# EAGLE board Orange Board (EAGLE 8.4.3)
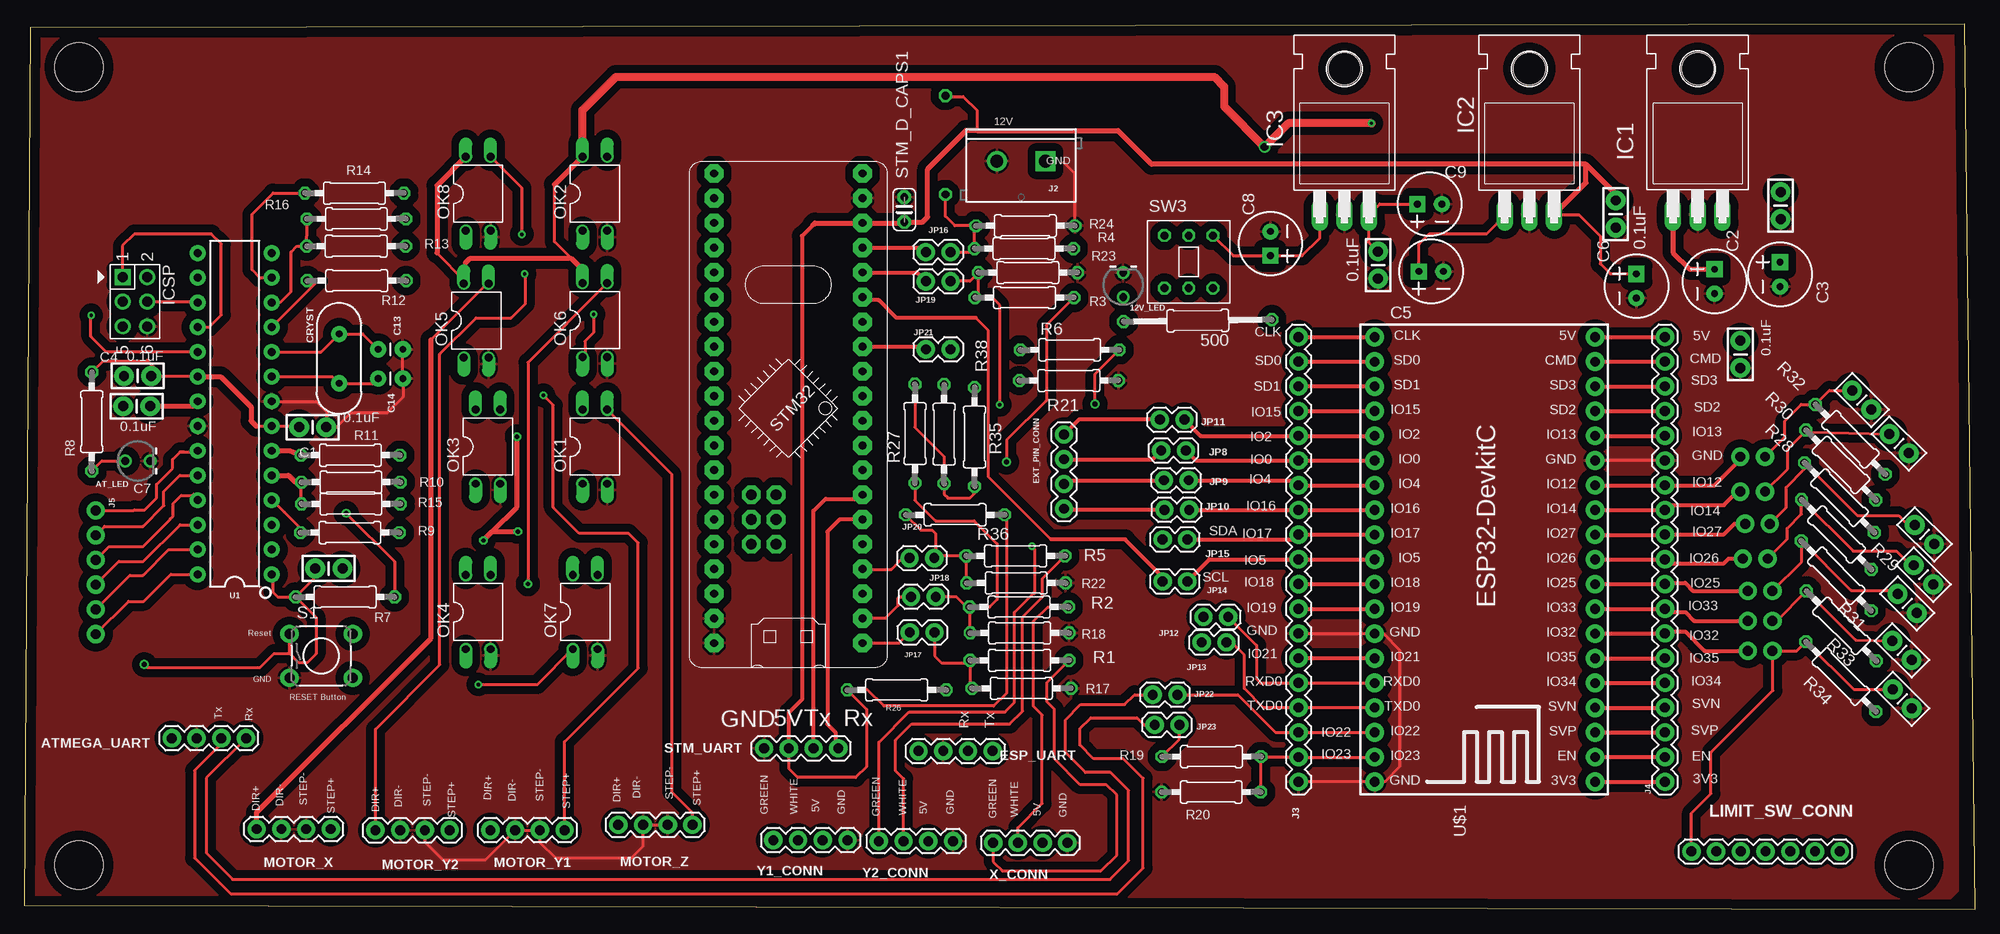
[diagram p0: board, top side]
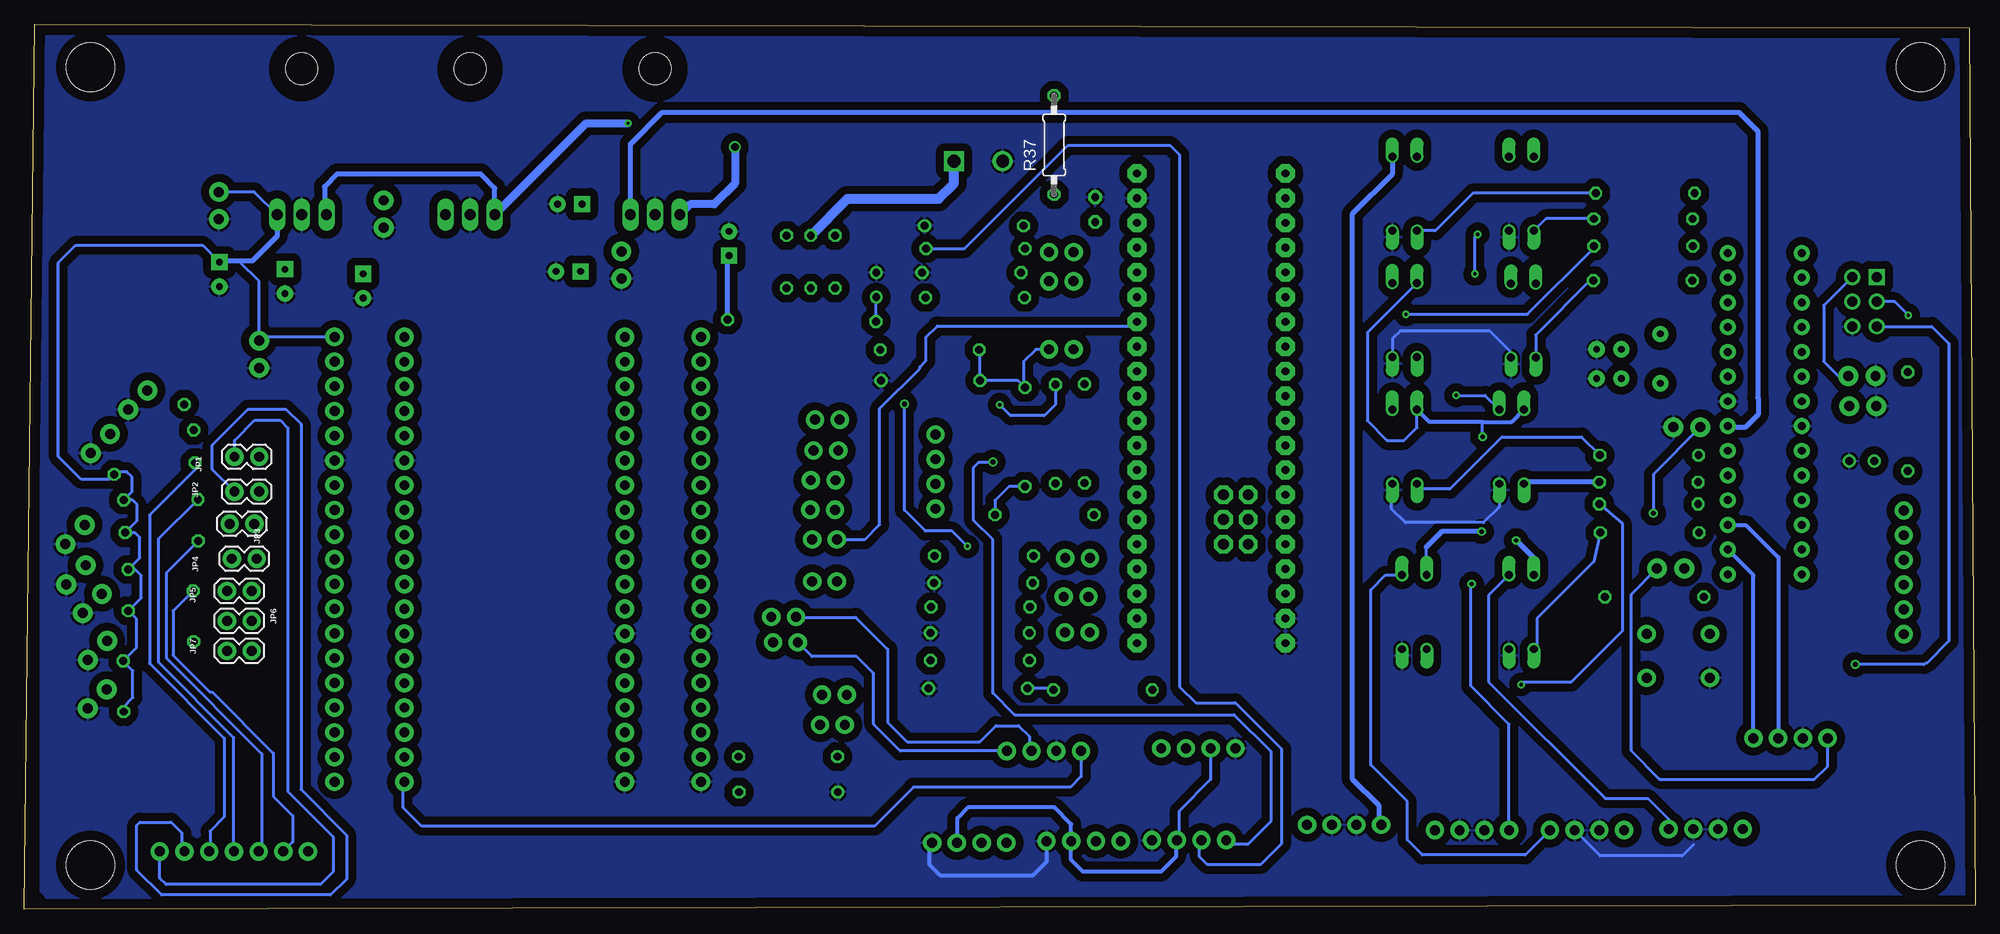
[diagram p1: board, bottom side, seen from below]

Size 200.42 x 90.95 mm. Coordinates in mm from the lower left corner, seen from the top.
Outline: 0,0.41 200.42,0 199.36,90.95 0.6,90.58 0,0.41
Copper layers (1*16): Top 0.035mm / dielectric 1.5mm / Bottom 0.035mm
Design rules "default *": minimum track width 12mil, minimum drill 0.35mm, track to track 12mil, track to pad 12mil, pad to pad 12mil, via to via 12mil, smd to smd 6mil, copper to edge 40mil, drill to drill 12mil, minimum pad ring 10mil, minimum via ring 8mil, stop-mask expansion 4mil, vias tented up to drill 0mil, thermal gap 10mil
Holes 5 mm at 5.62,86.55 193.62,86.55 5.62,4.55 193.62,4.55

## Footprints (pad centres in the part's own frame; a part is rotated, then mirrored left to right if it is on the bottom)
LED_3MM-NS = drill 0.813: A -1.27,0; K 1.27,0
0207/15 = drill 0.813 octagon: 1 -7.62,0; 2 7.62,0
1X04 = drill 1.016 pad 1.88: 1 0,0; 2 2.54,0; 3 5.08,0; 4 7.62,0
CAP-PTH-SMALL-KIT = drill 1.016 pad 2.032: 1 -1.397,0; 2 1.397,0
CPOL-RADIAL-2.5MM-6.5MM = drill 0.7 pad 1.651 square: 1 1.25,0 | drill 0.7 pad 1.651: 2 -1.25,0
CAP-PTH-2.54 = drill 0.7 pad 1.651: 1 -1.27,0; 2 1.27,0
HC49US = drill 0.7 pad 1.651: 1 -2.54,0; 2 2.54,0
TO220H = drill 1.118 long: 1 -2.54,-10.16; 2 0,-10.16; 3 2.54,-10.16 | hole 3.302: 0,4.826
HEADER_PRG_2X03 = drill 1.02 pad 1.632 square: 1 -2.54,-1.27 | drill 1.02 pad 1.632: 2 -2.54,1.27; 3 0,-1.27; 4 0,1.27; 5 2.54,-1.27; 6 2.54,1.27
SCREWTERMINAL-5MM-2 = drill 1.3 pad 2.032 square: 1 0,0 | drill 1.3 pad 2.032: 2 5,0
1X19 = drill 1.016 pad 1.88: 1 0,0; 2 2.54,0; 3 5.08,0; 4 7.62,0; 5 10.16,0; 6 12.7,0; 7 15.24,0; 8 17.78,0; 9 20.32,0; 10 22.86,0; 11 25.4,0; 12 27.94,0; 13 30.48,0; 14 33.02,0; 15 35.56,0; 16 38.1,0; 17 40.64,0; 18 43.18,0; 19 45.72,0
1X06_NO_SILK = drill 1.016 pad 1.88: 1 0,0; 2 2.54,0; 3 5.08,0; 4 7.62,0; 5 10.16,0; 6 12.7,0
1X02 = drill 1.016 pad 1.88: 1 0,0; 2 2.54,0
1X07 = drill 1.016 pad 1.88: 1 0,0; 2 2.54,0; 3 5.08,0; 4 7.62,0; 5 10.16,0; 6 12.7,0; 7 15.24,0
DIL04 = drill 0.813 offset: 1 -1.27,-3.81; 2 1.27,-3.81; 3 1.27,3.81; 4 -1.27,3.81
0207/10 = drill 0.813 octagon: 1 -5.08,0; 2 5.08,0
TACTILE-PTH = drill 1.016 pad 1.88: 1 -3.251,2.261; 2 3.251,2.261; 3 -3.251,-2.261; 4 3.251,-2.261
C025-024X044 = drill 0.813 pad 1.422 octagon: 1 -1.27,0; 2 1.27,0
SW_PUSH_BUTTON_MINI = drill 0.8 octagon: 1 2.5,2.7; 2 0,2.7; 3 -2.5,2.7; 4 2.5,-2.7; 5 0,-2.7; 6 -2.5,-2.7
DIP28 = drill 0.813 pad 1.626: 1 -16.51,-3.81; 2 -13.97,-3.81; 3 -11.43,-3.81; 4 -8.89,-3.81; 5 -6.35,-3.81; 6 -3.81,-3.81; 7 -1.27,-3.81; 8 1.27,-3.81; 9 3.81,-3.81; 10 6.35,-3.81; 11 8.89,-3.81; 12 11.43,-3.81; 13 13.97,-3.81; 14 16.51,-3.81; 15 16.51,3.81; 16 13.97,3.81; 17 11.43,3.81; 18 8.89,3.81; 19 6.35,3.81; 20 3.81,3.81; 21 1.27,3.81; 22 -1.27,3.81; 23 -3.81,3.81; 24 -6.35,3.81; 25 -8.89,3.81; 26 -11.43,3.81; 27 -13.97,3.81; 28 -16.51,3.81
ESP32-DEVKITC = drill 1 pad 1.93: 1 -22.87,-11.42; 2 -20.33,-11.42; 3 -17.79,-11.42; 4 -15.25,-11.42; 5 -12.71,-11.42; 6 -10.17,-11.42; 7 -7.63,-11.42; 8 -5.09,-11.42; 9 -2.55,-11.42; 10 -0.01,-11.42; 11 2.53,-11.42; 12 5.07,-11.42; 13 7.61,-11.42; 14 10.15,-11.42; 15 12.69,-11.42; 16 15.23,-11.42; 17 17.77,-11.42; 18 20.31,-11.42; 19 22.85,-11.42; 20 22.85,11.23; 21 20.31,11.23; 22 17.77,11.23; 23 15.23,11.23; 24 12.69,11.23; 25 10.15,11.23; 26 7.61,11.23; 27 5.07,11.23; 28 2.53,11.23; 29 -0.01,11.23; 30 -2.55,11.23; 31 -5.09,11.23; 32 -7.63,11.23; 33 -10.17,11.23; 34 -12.71,11.23; 35 -15.25,11.23; 36 -17.79,11.23; 37 -20.33,11.23; 38 -22.87,11.23
BLUE_PILL_ADV = drill 0.8 pad 1.93 octagon: P$1 10.16,-30.48; P$2 10.16,-27.94; P$3 10.16,-25.4; P$4 10.16,-22.86; P$5 10.16,-20.32; P$6 10.16,-17.78; P$7 10.16,-15.24; P$8 10.16,-12.7; P$9 10.16,-10.16; P$10 10.16,-7.62; P$11 10.16,-5.08; P$12 10.16,-2.54; P$13 10.16,0; P$14 10.16,2.54; P$15 10.16,5.08; P$16 10.16,7.62; P$17 10.16,10.16; P$18 10.16,12.7; P$19 10.16,15.24; P$20 10.16,17.78; P$21 -5.08,-30.48; P$22 -5.08,-27.94; P$23 -5.08,-25.4; P$24 -5.08,-22.86; P$25 -5.08,-20.32; P$26 -5.08,-17.78; P$27 -5.08,-15.24; P$28 -5.08,-12.7; P$29 -5.08,-10.16; P$30 -5.08,-7.62; P$31 -5.08,-5.08; P$32 -5.08,-2.54; P$33 -5.08,0; P$34 -5.08,2.54; P$35 -5.08,5.08; P$36 -5.08,7.62; P$37 -5.08,10.16; P$38 -5.08,12.7; P$39 -5.08,15.24; P$40 -5.08,17.78 | drill 1.1 pad 1.93 octagon: P$42 -1.27,-20.32; P$43 -1.27,-17.78; P$44 -1.27,-15.24; P$45 1.27,-15.24; P$46 1.27,-17.78; P$47 1.27,-20.32

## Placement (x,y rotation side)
12V_LED  [LED_3MM-NS]  112.9,64.18 90 top
500  1K  [0207/15]  120.55,60.5 180.7 top
AT_LED  [LED_3MM-NS]  11.65,46.08 0 top
ATMEGA_UART  [1X04]  22.78,17.59 180 top
C1  0.1uF  [CAP-PTH-SMALL-KIT]  29.62,49.55 0 top
C2  100uF  [CPOL-RADIAL-2.5MM-6.5MM]  173.65,64.53 90 top
C3  100uF  [CPOL-RADIAL-2.5MM-6.5MM]  180.38,65.25 90 top
C4  0.1uF  [CAP-PTH-SMALL-KIT]  11.63,54.82 180 top
C5  100uF  [CPOL-RADIAL-2.5MM-6.5MM]  144.53,65.56 180 top
C6  100uF  [CPOL-RADIAL-2.5MM-6.5MM]  165.63,64.06 90 top
C7  0.1uF  [CAP-PTH-SMALL-KIT]  11.55,51.71 180 top
C8  100uF  [CPOL-RADIAL-2.5MM-6.5MM]  128.01,68.42 270 top
C9  100uF  [CPOL-RADIAL-2.5MM-6.5MM]  144.38,72.47 180 top
C10  0.1uF  [CAP-PTH-SMALL-KIT]  180.44,72.33 270 top
C11  0.1uF  [CAP-PTH-SMALL-KIT]  163.49,71.45 270 top
C12  0.1uF  [CAP-PTH-SMALL-KIT]  139.08,66.21 270 top
C13  22pF  [CAP-PTH-2.54]  37.62,57.55 180 top
C14  22pF  [CAP-PTH-2.54]  37.62,54.55 180 top
C15  0.1uF  [CAP-PTH-SMALL-KIT]  31.29,35.02 0 top
C18  0.1uF  [CAP-PTH-SMALL-KIT]  195.22,38.52 135 top
C19  0.1uF  [CAP-PTH-SMALL-KIT]  195.12,34.38 135 top
C20  0.1uF  [CAP-PTH-SMALL-KIT]  192.6,47.87 135 top
C21  0.1uF  [CAP-PTH-SMALL-KIT]  193.44,31.43 135 top
C22  0.1uF  [CAP-PTH-SMALL-KIT]  188.77,52.34 135 top
C23  0.1uF  [CAP-PTH-SMALL-KIT]  192.91,26.61 135 top
C24  0.1uF  [CAP-PTH-SMALL-KIT]  192.93,21.63 135 top
CRYST  16MHz  [HC49US]  32.33,56.6 270 top
ESP_D_CAPS  0.1uF  [CAP-PTH-SMALL-KIT]  176.3,57.04 270 top
ESP_UART  [1X04]  99.48,16.27 180 top
EXT_PIN_CONN  [1X04]  106.81,41.17 90 top
IC1  7805T  [TO220H]  171.92,81.56 0 top
IC2  7805T  [TO220H]  154.62,81.55 0 top
IC3  7805T  [TO220H]  135.62,81.55 0 top
ICSP  CON_HEADER_PRG_AVR_ICSP-PTH  [HEADER_PRG_2X03]  11.36,62.45 270 top
J2  [SCREWTERMINAL-5MM-2]  104.92,76.89 180 top
J3  [1X19]  130.91,13.11 90 top
J4  [1X19]  168.55,13.11 90 top
J5  [1X06_NO_SILK]  7.33,40.99 270 top
JP1  [1X02]  176.29,46.51 180 bottom
JP2  [1X02]  176.29,42.93 180 bottom
JP3  [1X02]  176.79,39.62 180 bottom
JP4  [1X02]  176.56,36.04 180 bottom
JP5  [1X02]  177.06,32.73 180 bottom
JP6  [1X02]  177.06,29.65 180 bottom
JP7  [1X02]  177.06,26.57 180 bottom
JP8  [1X02]  119.34,47.16 180 top
JP9  [1X02]  119.62,44.09 180 top
JP10  [1X02]  119.67,41.06 180 top
JP11  [1X02]  119.19,50.32 180 top
JP12  [1X02]  123.68,30.05 180 top
JP13  [1X02]  123.5,27.44 180 top
JP14  [1X02]  119.48,33.7 180 top
JP15  [1X02]  119.48,38.01 180 top
JP16  [1X02]  92.62,67.55 0 top
JP17  [1X02]  90.97,28.45 0 top
JP18  [1X02]  91.1,32.12 0 top
JP19  [1X02]  92.62,64.55 0 top
JP20  [1X02]  90.94,36.1 0 top
JP21  [1X02]  92.62,57.55 0 top
JP22  [1X02]  118.47,22.06 180 top
JP23  [1X02]  118.67,18.96 180 top
LIMIT_SW_CONN  [1X07]  186.51,5.95 180 top
MOTOR_X  [1X04]  31.49,8.25 180 top
MOTOR_Y1  [1X04]  55.5,8.14 180 top
MOTOR_Y2  [1X04]  43.69,8.13 180 top
MOTOR_Z  [1X04]  68.64,8.69 180 top
OK1  PC817  [DIL04]  58.62,47.55 0 top
OK2  PC817  [DIL04]  58.62,73.55 0 top
OK3  PC817  [DIL04]  47.62,47.55 0 top
OK4  PC817  [DIL04]  46.62,30.55 0 top
OK5  PC817  [DIL04]  46.42,60.51 0 top
OK6  PC817  [DIL04]  58.62,60.55 0 top
OK7  PC817  [DIL04]  57.62,30.55 0 top
OK8  PC817  [DIL04]  46.62,73.55 0 top
R1  1K  [0207/10]  102.25,25.58 0 top
R2  1K  [0207/10]  102.19,31.07 0 top
R3  1K  [0207/10]  102.75,62.87 0 top
R4  1K  [0207/10]  102.7,67.91 0 top
R5  1K  [0207/10]  101.84,36.33 0 top
R6  1K  [0207/10]  107.4,57.5 0 top
R7  1K  [0207/10]  32.95,32.11 0 top
R8  1K  [0207/10]  6.93,50.12 270 top
R9  1K  [0207/10]  33.44,38.71 0 top
R10  1K  [0207/10]  33.55,43.9 0 top
R11  1K  [0207/10]  33.5,46.67 0 top
R12  1K  [0207/10]  34.15,64.61 0 top
R13  1K  [0207/10]  34.09,68.15 0 top
R14  1K  [0207/10]  33.91,73.61 0 top
R15  1K  [0207/10]  33.55,41.66 0 top
R16  1K  [0207/10]  34.11,70.96 0 top
R17  2K  [0207/10]  102.43,22.71 180 top
R18  2K  [0207/10]  102.25,28.41 180 top
R19  1K  [0207/10]  121.97,15.7 0 top
R20  1K  [0207/10]  121.93,12.05 180 top
R21  2K  [0207/10]  107.32,54.35 180 top
R22  2K  [0207/10]  101.9,33.53 180 top
R23  2K  [0207/10]  103.1,65.44 180 top
R24  2K  [0207/10]  102.84,70.24 180 top
R26  1K  [0207/10]  89.62,22.55 180 top
R27  1K  [0207/10]  91.5,48.89 90 top
R28  [0207/10]  186.48,42.31 135 top
R29  [0207/10]  186.17,38.52 135 top
R30  [0207/10]  186.63,45.66 135 top
R31  [0207/10]  186.15,34.28 135 top
R32  [0207/10]  187.6,48.3 135 top
R33  [0207/10]  186.68,29.12 135 top
R34  [0207/10]  186.63,23.92 135 top
R35  1K  [0207/10]  97.62,48.55 270 top
R36  1K  [0207/10]  95.62,40.55 0 top
R37  1K  [0207/10]  94.62,78.55 90 bottom
R38  1K  [0207/10]  94.5,48.84 270 top
S1  [TACTILE-PTH]  30.5,26.05 0 top
STM_D_CAPS1  0.1uF  [C025-024X044]  90.41,71.91 90 top
STM_UART  [1X04]  83.62,16.55 180 top
SW3  SW_PUSH_DPDT  [SW_PUSH_BUTTON_MINI]  119.62,66.55 0 top
U1  328P  [DIP28]  21.61,50.94 90 top
U$1  ESP32DEVKITC  [ESP32-DEVKITC]  149.96,35.97 90 top
U$2  [BLUE_PILL_ADV]  75.95,57.84 0 top
X_CONN  [1X04]  99.53,6.84 0 top
Y1_CONN  [1X04]  76.94,7.11 0 top
Y2_CONN  [1X04]  87.79,7.01 0 top

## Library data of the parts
12V_LED AT_LED = SparkFun-LED
500 R1-R24 R26-R38 = resistor
ATMEGA_UART ESP_UART EXT_PIN_CONN MOTOR_X MOTOR_Y1 MOTOR_Y2 MOTOR_Z STM_UART X_CONN Y1_CONN Y2_CONN = SparkFun-Connectors; PROD_ID: CONN-09696
C1 C4 C7 C10-C12 C15 C18-C24 ESP_D_CAPS = SparkFun-Capacitors; PROD_ID: CAP-08370
C2 C3 C5 C6 C8 C9 = SparkFun-Capacitors; PROD_ID: CAP-08439
C13 C14 = SparkFun-Capacitors; PROD_ID: CAP-09128
CRYST = SparkFun-Clocks; PROD_ID: XTAL-08181; SF_ID: COM-00536
IC1-IC3 STM_D_CAPS1 = adafruit
ICSP SW3 = dp_devices
J2 = SparkFun-Connectors; SF_SKU: PRT-08432
J3 J4 LIMIT_SW_CONN = SparkFun-Connectors
J5 = SparkFun-Connectors; PROD_ID: CONN-08437
JP1-JP23 S1 = SparkFun-Retired
OK1-OK8 = optocoupler; MPN: PC817X4J000F; OC_FARNELL: 9707727; OC_NEWARK: 97K7059
U1 = SparkFun-IC-Microcontroller; PROD_ID: IC-09136
U$1 = ESP32-DEVKITC
U$2 = BluePill

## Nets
3V3: ESP_UART.4 J4.1 U$1.1
12V: J2.1 SW3.2
12V_SIN: 500.1 C2.1 C5.1 C8.1 IC1.1 IC2.1 IC3.1 OK1.4 OK2.4 OK3.4 OK4.4 OK5.4 OK6.4 OK7.4 OK8.4 SW3.1
A0: J5.1 U1.23
A1: J5.2 U1.24
A2: J5.3 U1.25
A3: J5.4 U1.26
A4: J5.5 U1.27
A5: J5.6 U1.28
AT_5V: C1.1 C4.1 C9.1 C12.1 IC3.3 ICSP.2 R7.2 R8.1 U1.7 U1.20
AT_JRX: ATMEGA_UART.1 JP22.2 U1.2
AT_JTX: ATMEGA_UART.2 JP23.2 U1.3
AT_MISO: ICSP.1 U1.18
AT_MOSI: ICSP.4 U1.17
AT_RESET: C15.1 ICSP.5 R7.1 S1.1 U1.1
AT_RX: J3.3 JP22.1 U$1.36
AT_SCK: ICSP.3 U1.19
AT_SS: U1.16
AT_TX: J3.2 R19.2 R20.1 U$1.37
CLK: J3.19 U$1.20
CMD: J4.18 U$1.18
DIR_X: R12.1 U1.11
DIR_XO: MOTOR_X.4 OK5.3
DIR_Y: R13.1 R16.1 U1.12
DIR_Y1O: MOTOR_Y1.4 OK6.3
DIR_Y2O: MOTOR_Y2.4 OK8.3
DIR_Z: R14.1 U1.13
DIR_ZO: MOTOR_Z.4 OK2.3
DTR: ATMEGA_UART.4 C15.2
EN: J4.2 U$1.2
ENC_X_GR: JP19.1 U$2.P$16
ENC_X_JGR: R3.2 Y1_CONN.1
ENC_X_JWH: R4.2 Y1_CONN.2
ENC_X_WH: JP16.1 U$2.P$17
ENC_Y1_GR: JP17.1 U$2.P$1
ENC_Y1_JGR: R1.2 X_CONN.1
ENC_Y1_JWH: R2.2 X_CONN.2
ENC_Y1_WH: JP18.1 U$2.P$2
ENC_Y2_GR: JP21.1 U$2.P$13
ENC_Y2_JGR: R6.2 Y2_CONN.1
ENC_Y2_JWH: R5.2 Y2_CONN.2
ENC_Y2_WH: JP20.1 U$2.P$4
ESP32_5V: C3.1 C10.1 ESP_D_CAPS.1 IC1.3 J4.19 R28.1 R29.1 R30.1 R31.1 R32.1 R33.1 R34.1 U$1.19
ESP32_I2C_JSCL: JP14.2 U$2.P$15
ESP32_I2C_JSDA: JP15.2 U$2.P$14
ESP32_I2C_SCL: J3.10 JP14.1 U$1.29
ESP32_I2C_SDA: J3.11 JP15.1 U$1.28
ESP32_JRX: ESP_UART.2 JP12.2
ESP32_JTX: ESP_UART.1 JP13.2
ESP32_RX: J3.5 JP12.1 U$1.34
ESP32_TX: J3.4 JP13.1 U$1.35
EXT_P1: J3.15 JP11.1 U$1.24
EXT_P2: J3.14 JP8.1 U$1.25
EXT_P3: J3.13 JP9.1 U$1.26
EXT_P4: J3.12 JP10.1 U$1.27
EXT_PJ1: EXT_PIN_CONN.4 JP11.2
EXT_PJ2: EXT_PIN_CONN.3 JP8.2
EXT_PJ3: EXT_PIN_CONN.2 JP9.2
EXT_PJ4: EXT_PIN_CONN.1 JP10.2
GND: 12V_LED.K AT_LED.K ATMEGA_UART.3 C1.2 C2.2 C3.2 C4.2 C5.2 C6.2 C7.2 C8.2 C9.2 C10.2 C11.2 C12.2 C13.1 C14.1 C18.1 C19.1 C20.1 C21.1 C22.1 C23.1 C24.1 ESP_D_CAPS.2 ESP_UART.3 IC1.2 IC2.2 IC3.2 ICSP.6 J2.2 J3.1 J3.7 J4.14 MOTOR_X.2 MOTOR_X.3 MOTOR_Y1.2 MOTOR_Y1.3 MOTOR_Y2.2 MOTOR_Y2.3 MOTOR_Z.2 MOTOR_Z.3 OK1.2 OK2.2 OK3.2 OK4.2 OK5.2 OK6.2 OK7.2 OK8.2 R17.1 R18.1 R20.2 R21.1 R22.1 R23.1 R24.1 S1.3 STM_D_CAPS1.2 STM_UART.4 U1.8 U1.22 U$1.14 U$1.32 U$1.38 U$2.P$19 U$2.P$21 U$2.P$22 X_CONN.4 Y1_CONN.4 Y2_CONN.4
IO13: J4.15 U$1.15
IO15: J3.16 U$1.23
IO18: J3.9 U$1.30
IO19: J3.8 U$1.31
IO21: J3.6 U$1.33
IO34: J4.5 U$1.5
IO35: J4.6 U$1.6
LIMIT_SW1: J4.13 JP1.1 U$1.13
LIMIT_SW2: J4.12 JP2.1 U$1.12
LIMIT_SW3: J4.11 JP3.1 U$1.11
LIMIT_SW4: J4.10 JP4.1 U$1.10
LIMIT_SW5: J4.9 JP5.1 U$1.9
LIMIT_SW6: J4.8 JP6.1 U$1.8
LIMIT_SW7: J4.7 JP7.1 U$1.7
LIMIT_SWJ1: C22.2 JP1.2 LIMIT_SW_CONN.1 R32.2
LIMIT_SWJ2: C20.2 JP2.2 LIMIT_SW_CONN.2 R30.2
LIMIT_SWJ3: C18.2 JP3.2 LIMIT_SW_CONN.3 R28.2
LIMIT_SWJ4: C19.2 JP4.2 LIMIT_SW_CONN.4 R29.2
LIMIT_SWJ5: C21.2 JP5.2 LIMIT_SW_CONN.5 R31.2
LIMIT_SWJ6: C23.2 JP6.2 LIMIT_SW_CONN.6 R33.2
LIMIT_SWJ7: C24.2 JP7.2 LIMIT_SW_CONN.7 R34.2
N$1: C13.2 CRYST.1 U1.10
N$2: C14.2 CRYST.2 U1.9
N$3: AT_LED.A R8.2
N$4: JP17.2 R1.1 R17.2 R26.1
N$5: C7.1 U1.21
N$6: OK4.1 R9.2
N$7: OK3.1 R10.2
N$8: OK1.1 R11.2
N$9: OK5.1 R12.2
N$10: OK2.1 R14.2
N$11: OK6.1 R13.2
N$12: OK7.1 R15.2
N$13: OK8.1 R16.2
N$14: JP19.2 R3.1 R23.2 R38.1
N$15: JP16.2 R4.1 R24.2 R37.1
N$16: JP23.1 R19.1
N$17: JP18.2 R2.1 R18.2 R27.1
N$18: JP21.2 R6.1 R21.2 R35.1
N$20: JP20.2 R5.1 R22.2 R36.1
N$22: 12V_LED.A 500.2
SD0: J3.18 U$1.21
SD1: J3.17 U$1.22
SD2: J4.16 U$1.16
SD3: J4.17 U$1.17
STEP_X: R9.1 U1.4
STEP_XO: MOTOR_X.1 OK4.3
STEP_Y: R10.1 R15.1 U1.5
STEP_Y1O: MOTOR_Y1.1 OK3.3
STEP_Y2O: MOTOR_Y2.1 OK7.3
STEP_Z: R11.1 U1.6
STEP_ZO: MOTOR_Z.1 OK1.3
STM_5V: C6.1 C11.1 IC2.3 R26.2 R27.2 R35.2 R36.2 R37.2 R38.2 STM_D_CAPS1.1 STM_UART.3 U$2.P$18 X_CONN.3 Y1_CONN.3 Y2_CONN.3
STM_RX: STM_UART.1 U$2.P$6
STM_TX: STM_UART.2 U$2.P$7
SVN: J4.4 U$1.4
SVP: J4.3 U$1.3

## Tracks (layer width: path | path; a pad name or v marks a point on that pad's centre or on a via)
3V3
  Top 0.406: U$1.1 J4.1
  Bottom 0.305: ESP_UART.4 91.86,13.65 92.96,12.56 109.09,12.56 113.1,8.55 159.58,8.55 161.48,10.45 161.48,12.99 U$1.1
12V
  Bottom 1.016: SW3.2 115.85,73.01 106.49,73.01 104.91,74.59 J2.1
12V_SIN  (via drill 0.35, 0.45, 0.81)
  Top 0.305: OK6.4 57.35,65.72 | SW3.1 124.2,67.17 C8.1 131.28,67.17 133.08,68.97 IC3.1 | 56.2,66.87 54.47,68.6 54.47,74.48 | 42.38,67.45 45.15,64.68 OK5.4 45.33,64.5 45.33,66.46 | C5.1 143.28,68.35 144.37,69.43 150.23,69.43 152.08,71.28 IC2.1
  Top 0.508: v47.16,37.91 48.07,38.83 | 48.07,38.83 v50.72,38.83 | 48.07,38.83 50.61,41.37 v50.61,48.58 | 57.35,65.72 56.2,66.87 45.74,66.87 45.33,66.46 | OK8.4 42.38,74.39 42.38,67.45 | 54.47,74.48 OK2.4 | IC1.1 169.38,67.51 171.11,65.78 C2.1
  Top 0.813: v138.4,80.79 129.86,80.79 v127.42,78.35 123.26,82.51 123.26,84.55 122.24,85.56 60.77,85.56 57.35,82.14 OK2.4
  Bottom 0.305: 56.41,37.2 56.41,34.42 OK7.4 | v50.61,48.58 50.61,50.1 | 151.51,70.82 IC2.1 | OK6.4 62.45,59.26 62.45,50.23 60.42,48.2 58.67,48.2 57.35,49.52 OK1.4
  Bottom 0.406: OK3.4 47.61,50.1 50.61,50.1 56.09,50.1 OK1.4
  Bottom 0.508: OK4.4 45.35,36.1 v47.16,37.91 | v50.72,38.83 54.78,38.83 56.41,37.2 | IC2.1 152.08,74.12 153.51,75.55 168.32,75.55 169.59,74.28 169.59,71.61 IC1.1 | 500.1 128.17,67 C8.1
  Bottom 0.813: IC2.1 142.68,80.79 v138.4,80.79 | v127.42,78.35 127.42,74.59 129.56,72.46 132.01,72.46 IC3.1
A0
  Top 0.305: 16.37,47.01 16.1,47.01 | 16.37,47.01 17.68,47.01 U1.23 | J5.1 11.22,40.99 11.29,41.06 12.39,41.06 13.58,42.26 13.58,43.68 15.23,45.33 15.23,46.24 15.99,47.01 16.37,47.01
A1
  Top 0.305: J5.2 8.25,39.36 12.21,39.36 14.34,41.49 14.34,42.97 15.97,44.59 U1.24
A2
  Top 0.305: J5.3 8.7,37.28 12.21,37.28 14.95,40.02 14.95,40.05 15.28,40.38 15.28,41.7 16.12,42.53 17.26,42.53 17.37,42.64 17.8,42.2 U1.25
A3
  Top 0.305: J5.4 9.72,35.75 12.23,35.75 15.99,39.51 U1.26
A4
  Top 0.305: J5.5 10.84,34.33 12.21,34.33 14.85,36.97 U1.27
A5
  Top 0.305: J5.6 10.71,31.66 12.29,31.66 15.05,34.43 U1.28
AT_5V  (via drill 0.51)
  Top 0.305: C1.1 28.1,49.67 U1.7 23.82,49.67 | U1.20 17.73,54.82 C4.1 13.35,55.15 13.35,55.67 12.62,56.4 12.56,56.35 8.08,56.35 R8.1 | C12.1 138.16,68.53 IC3.3 139.24,72.47 C9.1 | v33.06,40.71 38.03,35.74 R7.2
  Top 0.508: U1.20 20.16,54.75 23.28,51.63 23.28,50.21 23.82,49.67
  Bottom 0.305: ICSP.2 15.56,62.06 15.56,56.3 14.08,54.82 C4.1 | C1.1 33.06,44.71 v33.06,40.71
  Bottom 0.508: IC3.3 138.16,78.64 134.89,81.9 24.27,81.9 22.34,79.97 22.34,52.59 22.29,52.54 22.29,50.87 23.64,49.52 25.27,49.52 U1.7
AT_JRX
  Top 0.305: ATMEGA_UART.1 18.69,13.5 18.69,5.81 21.4,3.09 111.55,3.09 113.45,4.99 113.45,12.21 111.6,14.06 109.01,14.06 106.95,16.12 106.95,19.47 108.53,21.05 113.05,21.05 114.06,22.06 JP22.2
  Bottom 0.406: U1.2 22.76,34.31 22.78,34.29 ATMEGA_UART.1
AT_JTX
  Top 0.305: ATMEGA_UART.2 20.24,17.01 17.49,14.26 17.49,5.3 21.18,1.62 112.31,1.62 114.93,4.23 114.93,13.48 112.92,15.48 109.85,15.48 108.45,16.88 108.45,18.59 109.56,19.7 114.29,19.7 115.03,18.96 JP23.2
  Bottom 0.406: U1.3 25.35,39.44 23.49,39.44 20.22,36.17 20.22,17.61 ATMEGA_UART.2
AT_MISO
  Top 0.305: U1.18 18.99,59.83 20.24,61.08 20.24,68.39 19.22,69.41 11.29,69.41 10.08,68.19 10.08,65 ICSP.1
AT_MOSI
  Top 0.305: ICSP.4 17.72,62.45 U1.17
AT_RESET  (via drill 0.51)
  Top 0.305: U1.1 25.52,34.33 25.52,32.63 26.04,32.11 R7.1 | R7.1 29.89,34.12 C15.1 | R7.1 29.96,30.01 29.96,26.25 29.05,25.34 28.19,25.34 27.25,26.28 | v12.34,25.16 12.64,24.86 24.22,24.86 25.65,26.28 27.25,26.28 | 27.25,26.28 S1.1
  Bottom 0.305: ICSP.5 4.46,59.91 2.71,58.16 2.71,27.57 5,25.29 5.12,25.29 5.25,25.16 v12.34,25.16
AT_RX
  Top 0.305: 131.26,18.18 U$1.36 | 131.26,18.18 J3.3 | JP22.1 124.66,22.06 128.52,18.2 131.24,18.2 131.26,18.18
AT_SCK  (via drill 0.35)
  Top 0.305: ICSP.3 10.09,62.08 | v6.88,61.05 6.82,61 6.82,58.87 8.4,57.29 U1.19
  Bottom 0.305: v6.88,61.05 8.27,62.45 ICSP.3
AT_TX
  Top 0.305: R20.1 127.05,12.1 R19.2 127.1,15.65 J3.2 U$1.37
CLK
  Top 0.406: J3.19 U$1.20
CMD
  Top 0.406: U$1.18 J4.18
DIR_X
  Top 0.305: R12.1 30.2,64.61 U1.11
DIR_XO
  Top 0.305: 41.77,58.54 47.56,64.32 OK5.3
  Top 0.508: MOTOR_X.4 23.87,9.95 41.77,27.85 41.77,58.54
DIR_Y
  Top 0.305: R16.1 29.03,69.19 R13.1 27.99,68.15 27.4,67.56 27.4,63.46 26.3,62.37 U1.12
DIR_Y1O  (via drill 0.45)
  Top 0.305: v51.73,33.44 51.73,56.2 OK6.3
  Bottom 0.305: MOTOR_Y1.4 47.88,19.02 51.83,22.98 51.83,33.34 v51.73,33.44
DIR_Y2O  (via drill 0.35)
  Top 0.305: MOTOR_Y2.4 36.07,18.52 42.69,25.14 42.69,57.06 46.4,60.77 50,60.77 51.48,62.25 51.48,65.22 v51.4,65.29 | v51.12,69.38 51.12,74.13 OK8.3
  Bottom 0.305: v51.4,65.29 51.4,69.1 v51.12,69.38
DIR_Z
  Top 0.305: U1.13 25.37,64.86 24.25,64.86 23.39,65.72 23.39,71.44 25.55,73.61 R14.1
DIR_ZO
  Bottom 0.305: 61.28,8.95 MOTOR_Z.4
  Bottom 0.508: OK2.3 59.89,75.58 64.03,71.44 64.03,13.43 61.28,10.68 61.28,8.95
DTR
  Bottom 0.305: C15.2 35.37,32.33 35.37,16.32 32.43,13.38 16.5,13.38 15.16,14.72 ATMEGA_UART.4
EN
  Top 0.406: U$1.2 J4.2
ENC_X_GR
  Top 0.406: U$2.P$16 91.71,65.46 JP19.1
ENC_X_JGR  (via drill 0.51)
  Top 0.305: R3.2 105,60.04 105,52.31 100.91,48.22 v100.91,45.96
  Bottom 0.305: Y1_CONN.1 76.5,6.67 74.72,6.67 72.36,9.03 72.36,16.22 76.14,20 98.67,20 100.91,22.24 100.91,37.99 102.89,39.97 102.89,45.43 102.35,45.96 v100.91,45.96
ENC_X_JWH
  Bottom 0.305: R4.2 103.81,67.91 93.19,78.53 82.72,78.53 81.73,77.54 81.73,22.88 80.08,21.22 76.01,21.22 71.27,16.47 71.27,6.75 73.42,4.59 78.86,4.59 79.67,5.4 79.67,6.92 Y1_CONN.2
ENC_X_WH
  Top 0.406: U$2.P$17 92.17,68 JP16.1
ENC_Y1_GR
  Top 0.305: U$2.P$1 89.87,27.36 JP17.1
ENC_Y1_JGR
  Top 0.305: X_CONN.1 99.53,4.89 100.47,3.95 110.61,3.95 112.23,5.58 112.23,11.75 111.17,12.82 108.48,12.82 105.81,15.48 105.81,20.56 105.07,21.3 105.07,23.33 R1.2
ENC_Y1_JWH
  Top 0.305: X_CONN.2 102.07,8.4 104.56,10.89 104.56,19.98 103.7,20.84 103.7,29.63 105.14,31.07 R2.2
ENC_Y1_WH
  Top 0.305: U$2.P$2 86.15,29.94 88.49,29.94 89.78,31.23 89.78,31.94 89.96,32.12 JP18.1
ENC_Y2_GR
  Top 0.406: U$2.P$13 92.33,57.84 JP21.1
ENC_Y2_JGR  (via drill 0.35, 0.51)
  Top 0.305: Y2_CONN.1 87.79,17.17 90.9,20.28 100.75,20.28 101.72,21.25 101.72,30.52 103.67,32.48 103.83,32.48 103.83,37 v103.52,37.3 | v110,51.93 110,55.02 R6.2
  Bottom 0.305: v103.52,37.3 105.1,38.88 107.84,38.88 110,41.04 v110,51.93
ENC_Y2_JWH
  Top 0.305: Y2_CONN.2 90.33,13.41 89.53,14.21 89.53,17.41 91.15,19.04 101.24,19.04 102.56,20.36 102.56,30.06 104.59,32.1 104.59,34 R5.2
ENC_Y2_WH
  Top 0.305: U$2.P$4 86.15,34.94 89.07,34.94 90.23,36.1 JP20.1
ESP32_5V
  Top 0.406: U$1.19 J4.19 | 175.97,58.83 ESP_D_CAPS.1
  Bottom 0.305: R34.1 190.22,20.83 189.27,21.78 189.27,24.53 R33.1 188.92,26.89 188.89,26.89 188.89,29.84 R31.1 188.41,32.02 188.41,34.31 189.03,34.93 R29.1 188.56,36.13 188.56,38.22 189.06,38.71 R28.1 188.89,39.89 188.89,41.67 189.29,42.07 R30.1 189.35,42.94 189.35,44.41 189.88,44.95 190.95,44.95 R32.1 191.71,44.19 194.56,44.19 196.92,46.55 196.92,66.46 195.14,68.24 182.11,68.24 C3.1 180.34,66.54 178.3,66.54 176.3,64.54 ESP_D_CAPS.1 175.91,58.83 J4.19 | IC1.3 176.78,73.72 C10.1
  Bottom 0.508: IC1.3 174.46,69.18 177,66.64 180.24,66.64 C3.1
ESP32_I2C_JSCL
  Top 0.305: 105.48,38.01 99.05,44.44 99.05,59.48 97.76,60.77
  Top 0.406: JP14.2 116.94,34.17 113.1,38.01 105.48,38.01 | 97.76,60.77 89.63,60.77 87.8,62.6 86.43,62.6 U$2.P$15
ESP32_I2C_JSDA
  Bottom 0.305: JP15.2 114.07,38.01 112.54,39.54 112.54,51.48 108.42,55.59 108.42,55.74 107.79,56.38 107.79,58.79 106.62,59.96 86.53,59.96 U$2.P$14
ESP32_I2C_SCL
  Top 0.406: U$1.29 J3.10 121.75,35.97 JP14.1
ESP32_I2C_SDA
  Top 0.406: U$1.28 J3.11 130.41,38.01 JP15.1
ESP32_JRX
  Bottom 0.305: JP12.2 121.1,30.01 115,30.01 111.73,26.74 111.73,19.22 109.75,17.24 102.23,17.24 100.6,18.86 98.27,18.86 97.17,17.77 97.17,16.5 ESP_UART.2
ESP32_JTX
  Bottom 0.305: ESP_UART.1 110.43,16.27 113.18,19.01 113.18,24.25 114.9,25.97 119.5,25.97 JP13.2
ESP32_RX
  Top 0.305: JP12.1 126.59,27.14 126.59,23.66 126.98,23.27 J3.5 U$1.34
ESP32_TX
  Top 0.305: U$1.35 J3.4 127.31,20.73 125.34,22.7 125.34,26.13 124.03,27.44 JP13.1
EXT_P1
  Top 0.406: 131.08,48.66 U$1.24 | 131.08,48.66 J3.15 | JP11.1 120.85,48.66 131.08,48.66
EXT_P2
  Top 0.406: U$1.25 J3.14 120.37,46.13 JP8.1
EXT_P3
  Top 0.406: U$1.26 J3.13 130.41,44.09 JP9.1
EXT_P4
  Top 0.406: J3.12 | J3.12 U$1.27 | JP10.1 119.69,41.04 J3.12
EXT_PJ1
  Top 0.406: JP11.2 108.34,50.32 EXT_PIN_CONN.4
EXT_PJ2
  Top 0.406: EXT_PIN_CONN.3 115.89,46.25 JP8.2
EXT_PJ3
  Top 0.406: EXT_PIN_CONN.2 107.19,44.09 JP9.2
EXT_PJ4
  Top 0.406: JP10.2 106.92,41.06 EXT_PIN_CONN.1
GND
  Top 0.305: 176.04,55.38 ESP_D_CAPS.2 | J4.14 U$1.14 | J3.7 U$1.32 139.61,28.34 141.29,26.66 141.29,14.65 139.76,13.11 U$1.38 | U$1.38 J3.1 | U$1.38 | U1.8 29.97,52.21 31.08,51.09 31.08,49.61 C1.2 32.1,49.55 33.6,51.04 37.28,51.04 38.96,52.72 38.96,54.48 C14.1 C13.1 | MOTOR_Y2.2 41.15,6.94 42.99,5.1 47.37,5.1 MOTOR_Y1.3 MOTOR_Y1.2 52.96,6.91 54.58,5.3 62.4,5.3 63.62,6.52 63.56,6.58 MOTOR_Z.3 MOTOR_Z.2 | R24.1 107.92,75.62 106.8,76.75
  Bottom 0.305: OK3.2 48.89,41.36 50.51,39.74 58.54,39.74 59.96,41.16 59.96,43.67 OK1.2 | OK5.2 47.69,57.26 49.88,59.45 59.07,59.45 59.86,58.66 59.86,56.77 OK6.2 | 28.95,6.64 30.09,5.5 38.52,5.5 MOTOR_Y2.2
  Bottom 0.406: Y2_CONN.4 95.41,4.9 96.84,3.47 106.29,3.47 107.41,4.59 107.41,6.58 X_CONN.4
  pour Bottom (isolate 0.813): 1.77,0.85 0.73,1.89 0.73,1.97 0.73,89.52 1.29,90.08 198.44,90.08 198.8,89.73 198.8,1.84 197.81,0.85
  pour Top (isolate 0.813): 198.44,90.08 1.26,90.08 0.73,89.55 0.73,1.92 1.77,0.88 197.66,0.88 198.7,1.92 198.7,89.83
IO13
  Top 0.406: U$1.15 J4.15
IO15
  Top 0.406: J3.16 U$1.23
IO18
  Top 0.406: J3.9 U$1.30
IO19
  Top 0.406: J3.8 U$1.31
IO21
  Top 0.406: U$1.33 J3.6
IO34
  Top 0.406: U$1.5 J4.5
IO35
  Top 0.406: U$1.6 J4.6
LIMIT_SW1
  Top 0.406: U$1.13 J4.13 168.59,43.55 173.62,43.55 176.29,46.22 JP1.1
LIMIT_SW2
  Top 0.406: U$1.12 J4.12 169.05,41.55 174.62,41.55 176,42.93 JP2.1
LIMIT_SW3
  Top 0.406: U$1.11 J4.11 168.59,38.55 174.62,38.55 175.69,39.62 JP3.1
LIMIT_SW4
  Top 0.406: U$1.10 J4.10 168.97,35.55 174.62,35.55 175.11,36.04 JP4.1
LIMIT_SW5
  Top 0.406: U$1.9 J4.9 168.67,33.55 170.62,33.55 171.44,32.73 JP5.1
LIMIT_SW6
  Top 0.406: U$1.8 J4.8 168.89,30.55 170.62,30.55 171.52,29.65 JP6.1
LIMIT_SW7
  Top 0.406: U$1.7 J4.7 168.75,28.55 170.62,28.55 172.6,26.57 JP7.1
LIMIT_SWJ1
  Top 0.305: C22.2 185.44,53.33 R32.2 182.55,51.89 180.84,50.18 180.84,48.52 JP1.2
  Bottom 0.305: JP1.2 178.83,48.2 176.75,50.28 174.16,50.28 173.35,49.47 173.35,12.11 168.67,7.43 168.67,3.88 169.99,2.56 185.87,2.56 186.51,3.2 LIMIT_SW_CONN.1
LIMIT_SWJ2
  Top 0.305: C20.2 183.26,49.03 R30.2 183.04,49.15 181.17,47.28 181.17,45.27 JP2.2
  Bottom 0.305: JP2.2 181.12,45.22 181.12,47.72 177.44,51.4 173.55,51.4 172,49.85 172,12.31 167.33,7.64 167.33,3.11 168.97,1.48 186.31,1.48 188.87,4.03 188.87,8.65 188.56,8.96 185.34,8.96 184.24,7.86 184.24,6.23 LIMIT_SW_CONN.2
LIMIT_SWJ3
  Top 0.305: C18.2 193.42,39.59 192.55,40.45 188.33,40.45 R28.2 182.89,45.27 180.99,43.37 180.99,41.28 JP3.2
  Bottom 0.305: R28.2 182.89,45.19 187.55,40.53 187.55,25.26 179.88,17.59 179.88,9.51 181.35,8.04 181.35,6.04 LIMIT_SW_CONN.3
LIMIT_SWJ4
  Top 0.305: C19.2 193.77,35.37 192.32,36.82 187.88,36.82 R29.2 182.58,40.62 181.12,39.16 181.12,38.06 JP4.2
  Bottom 0.305: LIMIT_SW_CONN.4 178.89,17.65 186.61,25.36 186.61,38.09 R29.2
LIMIT_SWJ5
  Top 0.305: 182.59,37.84 R31.2 | 182.59,37.84 187.65,32.78 191.43,32.78 191.79,32.42 C21.2 | JP5.2 182.59,35.72 182.59,37.84
  Bottom 0.305: R31.2 185.84,34.58 185.84,25.82 176.01,15.99 176.01,6.29 LIMIT_SW_CONN.5
LIMIT_SWJ6
  Top 0.305: C23.2 188.11,27.7 R33.2 180.02,29.65 JP6.2
  Bottom 0.305: R33.2 | R33.2 185.13,30.67 185.13,26.1 181.37,22.34 181.15,22.34 174.85,16.04 174.85,11.62 172.84,9.62 172.84,6.93 LIMIT_SW_CONN.6
LIMIT_SWJ7
  Top 0.305: LIMIT_SW_CONN.7 171.27,9.88 173.27,11.88 173.27,16.12 179.65,22.49 179.65,26.52 JP7.2 182.1,26.57 R34.2 187.93,22.62 C24.2
N$1
  Top 0.305: U1.10 30.48,57.29 CRYST.1 34.76,59.14 C13.2
N$2
  Top 0.305: U1.9 31.64,54.75 CRYST.2 35.86,54.06 C14.2
N$3
  Top 0.305: R8.2 7.97,46.08 AT_LED.A
N$4
  Top 0.305: JP17.2 93.51,26.06 94.23,25.34 96.92,25.34 R1.1 97.17,22.9 R17.2
  Bottom 0.305: R26.1 94.86,22.71 R17.2
N$5
  Top 0.508: C7.1 17.3,51.71 U1.21
N$6
  Bottom 0.305: R9.2 39.16,35.75 45.03,29.89 45.03,27.06 OK4.1
N$7
  Bottom 0.508: R10.2 46.19,43.9 OK3.1
N$8
  Bottom 0.305: OK1.1 56.81,43.2 53.97,43.2 48.61,48.55 40.45,48.55 R11.2
N$9
  Bottom 0.305: R12.2 39.56,64.61 45.15,59.02 OK5.1
N$10
  Bottom 0.305: 54.3,70.91 54.07,71.14 | 54.3,70.91 55.46,69.74 OK2.1 | R14.2 51.59,73.61 54.3,70.91
N$11  (via drill 0.35)
  Top 0.305: v58.49,61.15 58.49,59.27 57.6,58.38 57.6,56.99 OK6.1
  Bottom 0.305: v58.49,61.15 45.99,61.15 39.17,67.98 R13.2
N$12  (via drill 0.35)
  Top 0.305: v46.65,23.1 52.71,23.1 OK7.1
  Bottom 0.305: R15.2 36.26,39.65 36.26,28.59 41.52,23.33 46.42,23.33 v46.65,23.1
N$13
  Bottom 0.305: R16.2 44.13,70.96 OK8.1
N$14  (via drill 0.35)
  Top 0.305: JP19.2 97.13,64.55 R23.2 98.02,63.22 R3.1 99.44,62.87 100.22,62.09 v100.22,51.86
  Bottom 0.305: R38.1 94.5,51.87 95.62,50.74 99.1,50.74 v100.22,51.86
N$15
  Top 0.305: JP16.2 97.27,67.55 R4.1 97.62,70.1 R24.2 95.6,70.24 94.62,71.22 R37.1
N$16
  Top 0.305: R19.1 118.67,17.48 JP23.1
N$17
  Top 0.305: R18.2 97.17,31.01 R2.1 | R2.1 96.8,31.07 95.75,32.12 JP18.2 | R27.1 91.5,42.04 93.62,39.92 97.58,39.92 99.94,37.56 99.94,31.84 99.17,31.07 R2.1
N$18
  Bottom 0.305: R6.1 102.23,57.41 R21.2 98.34,54.35 R35.1 97.76,53.77 97.76,56.3 96.51,57.55 JP21.2
N$20
  Top 0.305: R22.2 96.82,36.27 R5.1 93.71,36.33 93.61,36.22 | 93.61,36.22 JP20.2 | R36.1 92.11,38.98 93.26,38.98 93.61,38.63 93.61,36.22
N$22
  Bottom 0.305: 500.2 112.93,62.87 12V_LED.A
SD0
  Top 0.406: J3.18 U$1.21
SD1
  Top 0.406: U$1.22 J3.17
SD2
  Top 0.406: U$1.16 J4.16
SD3
  Top 0.406: U$1.17 J4.17
STEP_X
  Top 0.305: R9.1 28.36,39.16 26.73,40.79 | 26.73,40.79 26.66,40.86 | U1.4 25.47,42.05 26.73,40.79
STEP_XO
  Bottom 0.305: OK4.3 50,32.24 50,23.38 38.02,11.39 33.65,11.39 31.49,9.24 MOTOR_X.1
STEP_Y
  Top 0.305: 27.83,43.91 R10.1 R15.1
  Top 0.508: U1.5 27.15,44.59 27.83,43.91
STEP_Y1O  (via drill 0.35)
  Top 0.305: MOTOR_Y1.1 55.5,17.22 63.06,24.78 63.06,37.66 62.07,38.65 57.02,38.65 54.35,41.32 54.35,51.81 v53.33,52.82
  Bottom 0.305: v53.33,52.82 50.35,52.82 OK3.3
STEP_Y2O
  Bottom 0.305: MOTOR_Y2.1 46.22,5.6 56.81,5.6 58.34,7.13 58.34,11.09 62.09,14.85 62.09,32.83 60.57,34.36 OK7.3
STEP_Z
  Top 0.508: U1.6 27.27,47.13 R11.1
STEP_ZO
  Top 0.305: MOTOR_Z.1 68.64,9.93 66.54,12.03 66.54,44.71 OK1.3
STM_5V
  Top 0.305: IC2.3 159.71,71.39 161.89,69.2 161.89,66.33 162.92,65.31 C6.1 | 163.49,73.52 C11.1 | STM_UART.3 78.54,14.46 79.44,13.55 85.41,13.55 86.53,14.67 86.53,20.56 R26.2 86.65,22.55 88.31,20.89 99.59,20.89 100.91,22.21 100.91,40.34 R36.2 | R35.2 97.71,43.38 97.71,42.81 97.15,42.26 94.89,42.26 94.5,42.65 R38.2 94.5,46.53 91.5,49.53 R27.2 | R37.2 94.72,83.53 96.46,83.53 97.86,82.13 97.86,80.03
  Top 0.406: 81.01,70.33 79.88,69.2 79.88,21.55 78.54,20.22 STM_UART.3
  Top 0.508: 81.01,70.33 81.21,70.54 U$2.P$18 90.3,70.54 STM_D_CAPS1.1 92.28,70.64 92.8,71.16 92.8,76.09 96.74,80.03 97.86,80.03 112.36,80.03 115.82,76.57 160.44,76.57 | 157.6,70.95 IC2.3 160.44,74.67 160.44,76.57 | 160.44,76.57 163.49,73.52
  Bottom 0.152: X_CONN.3 104.56,6.89
  Bottom 0.305: STM_UART.3 78.54,13.34 81.78,10.1 81.78,7.35 Y1_CONN.3 | R35.2 99.26,43.47 100.7,42.03 R36.2
  Bottom 0.406: 104.56,6.89 104.56,9.36 103.45,10.48 94.61,10.48 92.87,8.74 Y2_CONN.3 92.87,5.08 91.66,3.88 83.63,3.88 82.11,5.4 82.11,7.02 Y1_CONN.3
STM_RX
  Top 0.406: U$2.P$6 83.75,40.06 82.52,38.83 82.52,19.01 83.33,18.2 83.33,16.84 STM_UART.1
STM_TX
  Top 0.406: STM_UART.2 81.08,40.95 82.31,42.18 85.69,42.18 U$2.P$7
SVN
  Top 0.406: U$1.4 J4.4
SVP
  Top 0.406: U$1.3 J4.3

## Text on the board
tNames: 12V | GND | 0.1uF | 0.1uF | CLK | 5V | C4 | 0.1uF | CMD | 0.1uF | SD0 | SD1 | SD3 | SD2 | IO15 | 0.1uF | 0.1uF | IO2 | IO13 | C1 | GND | IO0 | IO4 | IO12 | C7 | IO16 | IO14 | SDA | IO17 | IO27 | IO5 | IO26 | SCL | IO18 | IO25 | IO19 | IO33 | Reset | GND | IO32 | IO21 | IO35 | GND | RXD0 | IO34 | RESET Button | Rx | TXD0 | SVN | Tx | GND | 5V | Tx | Rx | Rx | Tx | IO22 | SVP | IO23 | EN | STEP+ | STEP+ | STEP+ | STEP+ | DIR+ | DIR+ | DIR+ | 3V3 | DIR+ | DIR- | STEP- | DIR- | STEP- | DIR- | STEP- | DIR- | STEP- | GREEN | WHITE | 5V | GND | GREEN | WHITE | 5V | GND | GREEN | WHITE | 5V | GND
tValues: 0.1uF | 0.1uF | 0.1uF | 0.1uF | 0.1uF | 0.1uF | DTS | GND | 0.1uF | GND
Notes: Reset | Fedd Hold | Cycle Start | Coolant EN | Reserved | Probe | 3.3V

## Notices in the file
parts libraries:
SparkFun-LED: Licensing: Creative Commons ShareAlike 4.0 International - https://creativecommons.org/licenses/by-sa/4.0
